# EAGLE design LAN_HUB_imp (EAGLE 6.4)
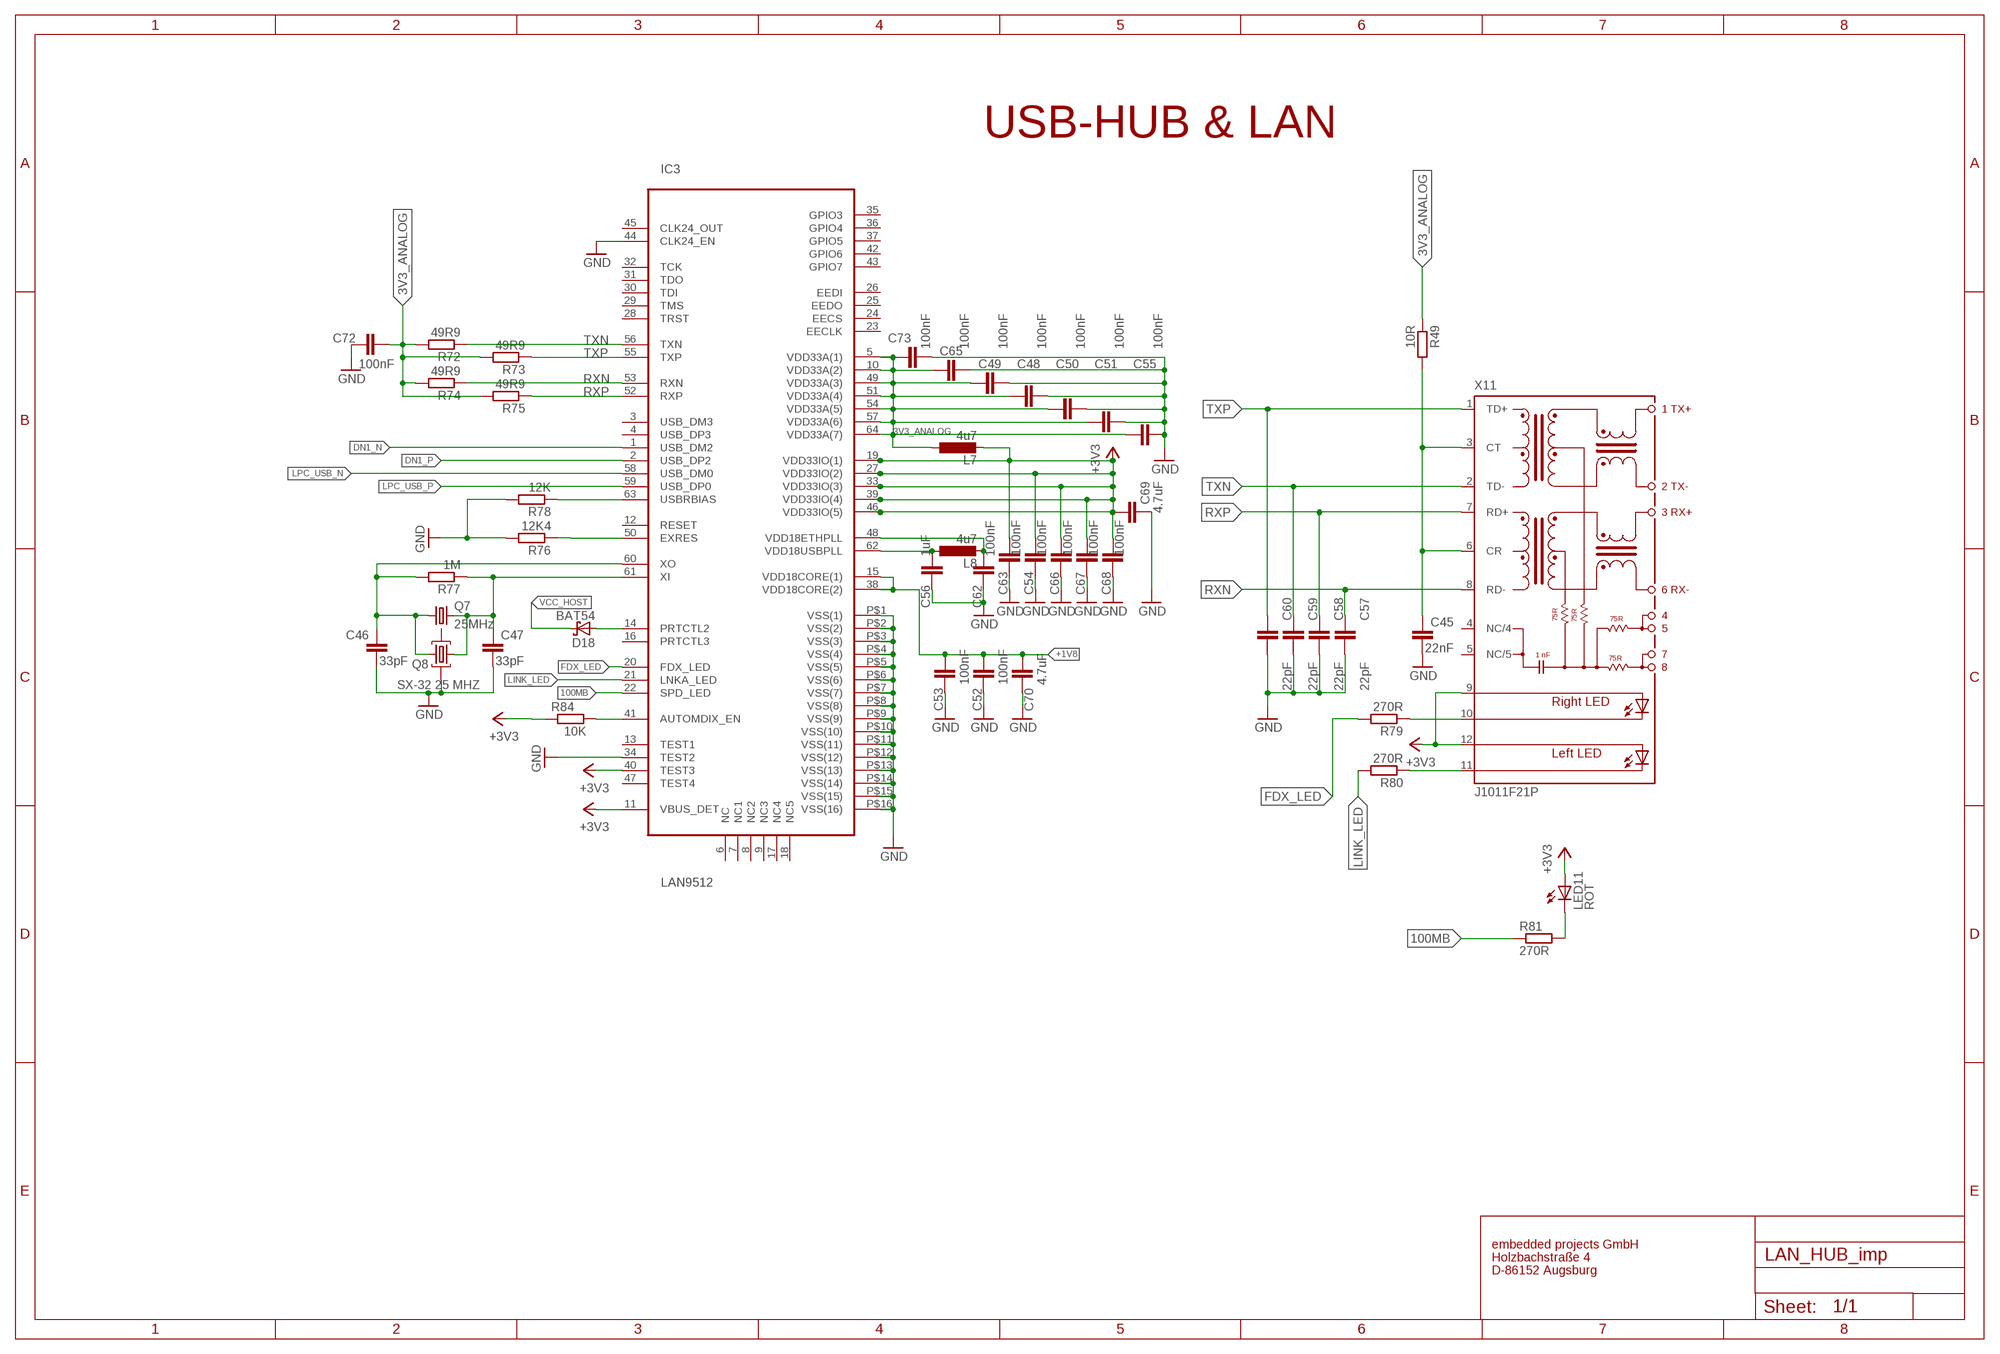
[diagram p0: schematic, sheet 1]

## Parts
C45  22nF  C-EUC0805  [C0805]
C46  33pF  C-EUC0805  [C0805]
C47  33pF  C-EUC0805  [C0805]
C48  100nF  C-EUC0805  [C0805]
C49  100nF  C-EUC0805  [C0805]
C50  100nF  C-EUC0805  [C0805]
C51  100nF  C-EUC0805  [C0805]
C52  100nF  C-EUC0805  [C0805]
C53  100nF  C-EUC0805  [C0805]
C54  100nF  C-EUC0805  [C0805]
C55  100nF  C-EUC0805  [C0805]
C56  1uF  C-EUC0805  [C0805]
C57  22pF  C-EUC0805  [C0805]
C58  22pF  C-EUC0805  [C0805]
C59  22pF  C-EUC0805  [C0805]
C60  22pF  C-EUC0805  [C0805]
C62  100nF  C-EUC0805  [C0805]
C63  100nF  C-EUC0805  [C0805]
C65  100nF  C-EUC0805  [C0805]
C66  100nF  C-EUC0805  [C0805]
C67  100nF  C-EUC0805  [C0805]
C68  100nF  C-EUC0805  [C0805]
C69  4.7uF  C-EUC0805  [C0805]
C70  4.7uF  C-EUC0805  [C0805]
C72  100nF  C-EUC0805  [C0805]
C73  100nF  C-EUC0805  [C0805]
D18  BAT54  DIODE_BAT54  [SOT-23]
IC3  LAN9512  [QFN-64]
L7  4u7  PSU3014  [PSU3014]
L8  4u7  PSU3014  [PSU3014]
LED11  ROT  LED_LEDCHIPLED_0805  [LED_CHIP-LED0805]
Q7  25MHz  CRYSTALHC49UP  [HC49UP]
Q8  SX-32 25 MHZ  SX-32  [SX-32]
R49  10R  R-EU_R0805  [R0805]
R72  49R9  R-EU_R0805  [R0805]
R73  49R9  R-EU_R0805  [R0805]
R74  49R9  R-EU_R0805  [R0805]
R75  49R9  R-EU_R0805  [R0805]
R76  12K4  R-EU_R0805  [R0805]
R77  1M  R-EU_R0805  [R0805]
R78  12K  R-EU_R0805  [R0805]
R79  270R  R-EU_R0805  [R0805]
R80  270R  R-EU_R0805  [R0805]
R81  270R  R-EU_R0805  [R0805]
R84  10K  R-EU_R0805  [R0805]
X11  J1011F21P  [J1]

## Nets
3V3_ANALOG: C48.2 C49.2 C50.2 C51.2 C55.2 C65.2 C72.1 C73.2 IC3.5(VDD33A(1)) IC3.10(VDD33A(2)) IC3.49(VDD33A(3)) IC3.51(VDD33A(4)) IC3.54(VDD33A(5)) IC3.57(VDD33A(6)) IC3.64(VDD33A(7)) L7.2 R49.1 R72.2 R73.2 R74.2 R75.2
100MB: IC3.22(SPD_LED) R81.1
+1V8: C52.2 C53.2 C70.1 IC3.15(VDD18CORE(1)) IC3.38(VDD18CORE(2))
+3V3: C54.2 C63.2 C66.2 C67.2 C68.2 C69.2 IC3.11(VBUS_DET) IC3.19(VDD33IO(1)) IC3.27(VDD33IO(2)) IC3.33(VDD33IO(3)) IC3.39(VDD33IO(4)) IC3.40(TEST3) IC3.46(VDD33IO(5)) L7.1 LED11.A R84.1 X11.9(A-R) X11.12(AL)
DN1_N: IC3.1(USB_DM2)
DN1_P: IC3.2(USB_DP2)
FDX_LED: IC3.20(FDX_LED) R79.2
GND: C45.1 C46.1 C47.1 C48.1 C49.1 C50.1 C51.1 C52.1 C53.1 C54.1 C55.1 C56.2 C57.1 C58.1 C59.1 C60.1 C62.2 C63.1 C65.1 C66.1 C67.1 C68.1 C69.1 C70.2 C72.2 C73.1 IC3.34(TEST2) IC3.44(CLK24_EN) IC3.P$1(VSS(1)) IC3.P$2(VSS(2)) IC3.P$3(VSS(3)) IC3.P$4(VSS(4)) IC3.P$5(VSS(5)) IC3.P$6(VSS(6)) IC3.P$7(VSS(7)) IC3.P$8(VSS(8)) IC3.P$9(VSS(9)) IC3.P$10(VSS(10)) IC3.P$11(VSS(11)) IC3.P$12(VSS(12)) IC3.P$13(VSS(13)) IC3.P$14(VSS(14)) IC3.P$15(VSS(15)) IC3.P$16(VSS(16)) Q8.2 R76.2 R78.2
LINK_LED: IC3.21(LNKA_LED) R80.2
LPC_USB_N: IC3.58(USB_DM0)
LPC_USB_P: IC3.59(USB_DP0)
N$10: C56.1 IC3.62(VDD18USBPLL) L8.2
N$11: LED11.C R81.2
N$21: C45.2 R49.2 X11.3(CT) X11.6(CR)
N$22: IC3.50(EXRES) R76.1
N$42: C62.1 IC3.48(VDD18ETHPLL) L8.1
N$61: C46.2 IC3.60(XO) Q7.1 Q8.3 R77.2
N$63: C47.2 IC3.61(XI) Q7.2 Q8.1 R77.1
N$65: IC3.63(USBRBIAS) R78.1
N$68: R79.1 X11.10(C-R)
N$76: R80.1 X11.11(C-L)
N$77: IC3.41(AUTOMDIX_EN) R84.2
N$78: D18.1(A) IC3.14(PRTCTL2)
RXN: C57.2 IC3.53(RXN) R74.1 X11.8(RD-)
RXP: C58.2 IC3.52(RXP) R75.1 X11.7(RD+)
TXN: C59.2 IC3.56(TXN) R72.1 X11.2(TD-)
TXP: C60.2 IC3.55(TXP) R73.1 X11.1(TD+)
VCC_HOST: D18.3(C)
Unconnected: IC3.3(USB_DM3) IC3.4(USB_DP3) IC3.6(NC) IC3.7(NC1) IC3.8(NC2) IC3.9(NC3) IC3.12(RESET) IC3.13(TEST1) IC3.16(PRTCTL3) IC3.17(NC4) IC3.18(NC5) IC3.23(EECLK) IC3.24(EECS) IC3.25(EEDO) IC3.26(EEDI) IC3.28(TRST) IC3.29(TMS) IC3.30(TDI) IC3.31(TDO) IC3.32(TCK) IC3.35(GPIO3) IC3.36(GPIO4) IC3.37(GPIO5) IC3.42(GPIO6) IC3.43(GPIO7) IC3.45(CLK24_OUT) IC3.47(TEST4) Q8.4 X11.4(NC/4) X11.5(NC/5)

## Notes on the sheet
- USB-HUB & LAN
- embedded projects GmbH
- Holzbachstraße 4
- D-86152 Augsburg

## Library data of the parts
C45-C60 C62 C63 C65-C70 C72 C73 = rcl:C-EU: CAPACITOR, European symbol
D18 = EmbeddedProjectsBauteile:DIODE_BAT54: Schottky Diodes; EP: 400113
IC3 = EmbeddedProjectsBauteile:LAN9512: USB 2.0 Hub and 10/100 Ethernet Controller; FARNELL: 2292586
L7 L8 = KUBUS3B_PARTS2:PSU3014: SMD Power Inductors Shielded
LED11 = EmbeddedProjectsBauteile:LED_LED
Q7 = crystal:CRYSTAL: CRYSTAL; OC_FARNELL: unknown; OC_NEWARK: unknown
Q8 = KUBUS3B_PARTS2:SX-32: SMD CRYSTAL; FARNELL: 1712841
R49 R72-R81 R84 = rcl:R-EU_: RESISTOR, European symbol
X11 = con-pulse:J1011F: PULSEJACK (TM) 1x1 Tab-UP RJ45 10/100 Base-TX RJ45 1x1 Tab-UP with LEDs 8-pin (J1 series) and 6-pin (JP series) integrated magnetics connector, designed to support applications, such as ADSL modems, LAN-on-Motherboard, and Hub and Switches. Source: www.pulseeng.com .. PulseJack-J402.pdf; OC_FARNELL: unknown; OC_NEWARK: unknown

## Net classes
0 default: clearance 0.15 mm
1 USB5V_EXT: width 0.15 mm, drill 0.3 mm, clearance 0.15 mm
2 5V: width 0.2 mm, clearance 0.15 mm
3 RELAY: width 1 mm, clearance 0.5 mm
5 0.15: width 0.125 mm, drill 0.3 mm, clearance 0.15 mm

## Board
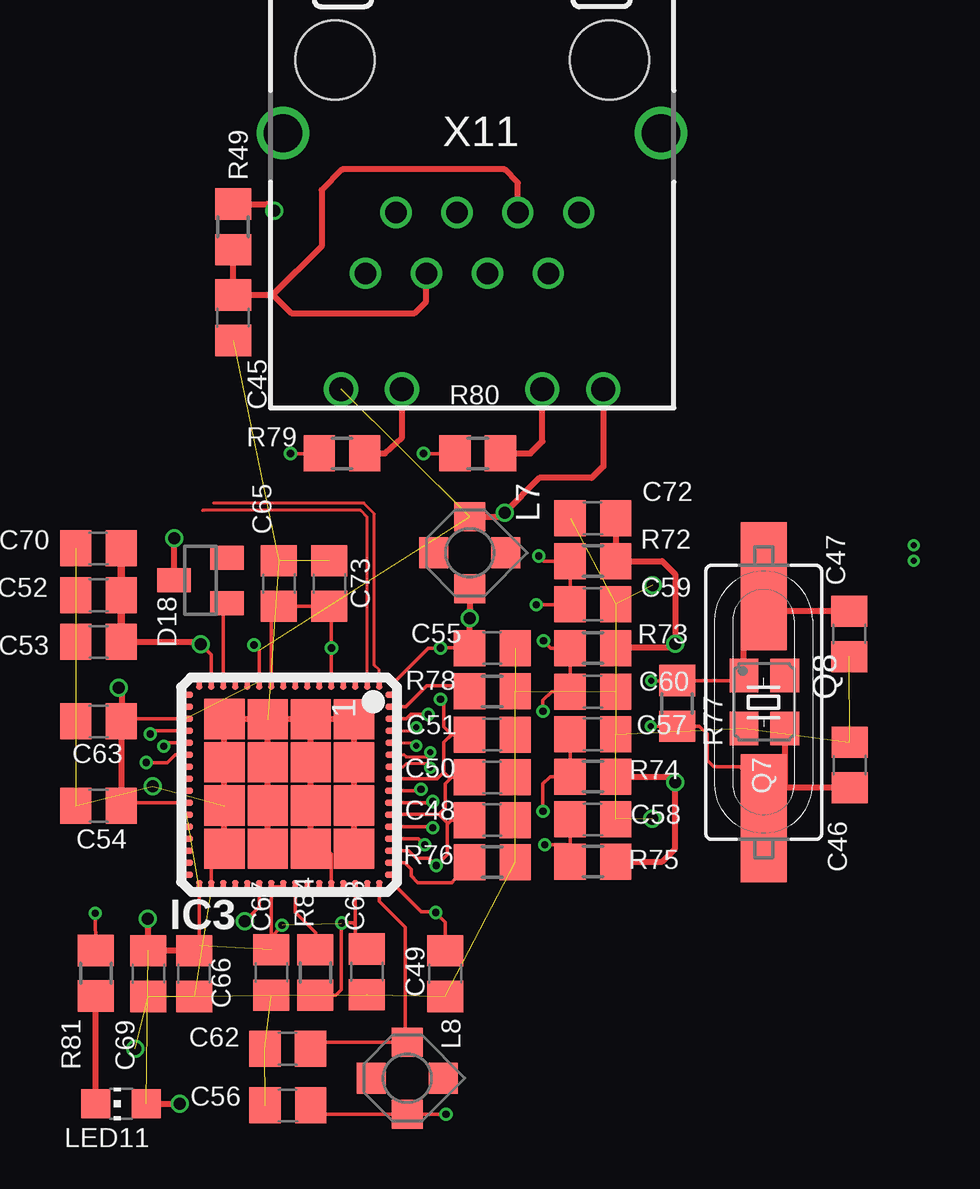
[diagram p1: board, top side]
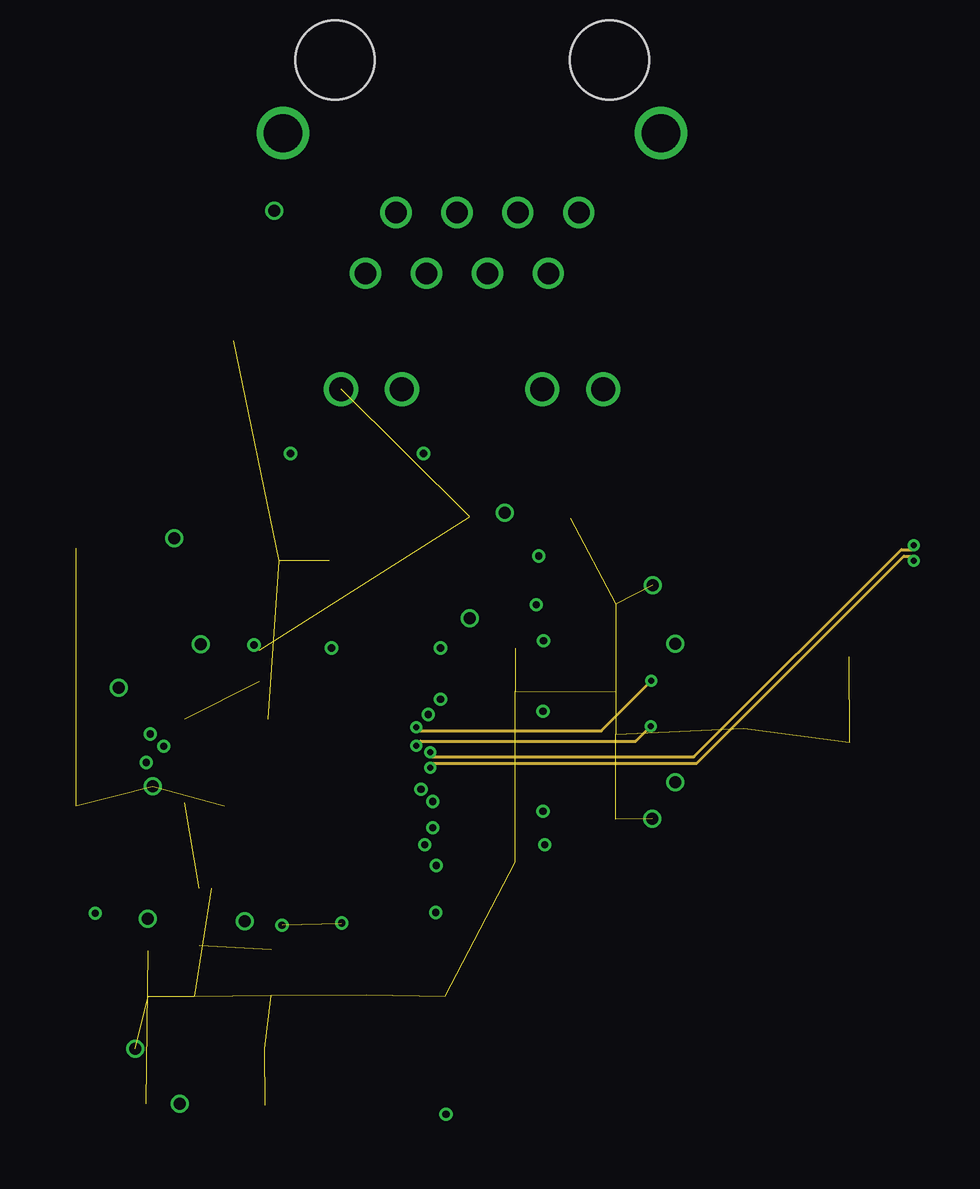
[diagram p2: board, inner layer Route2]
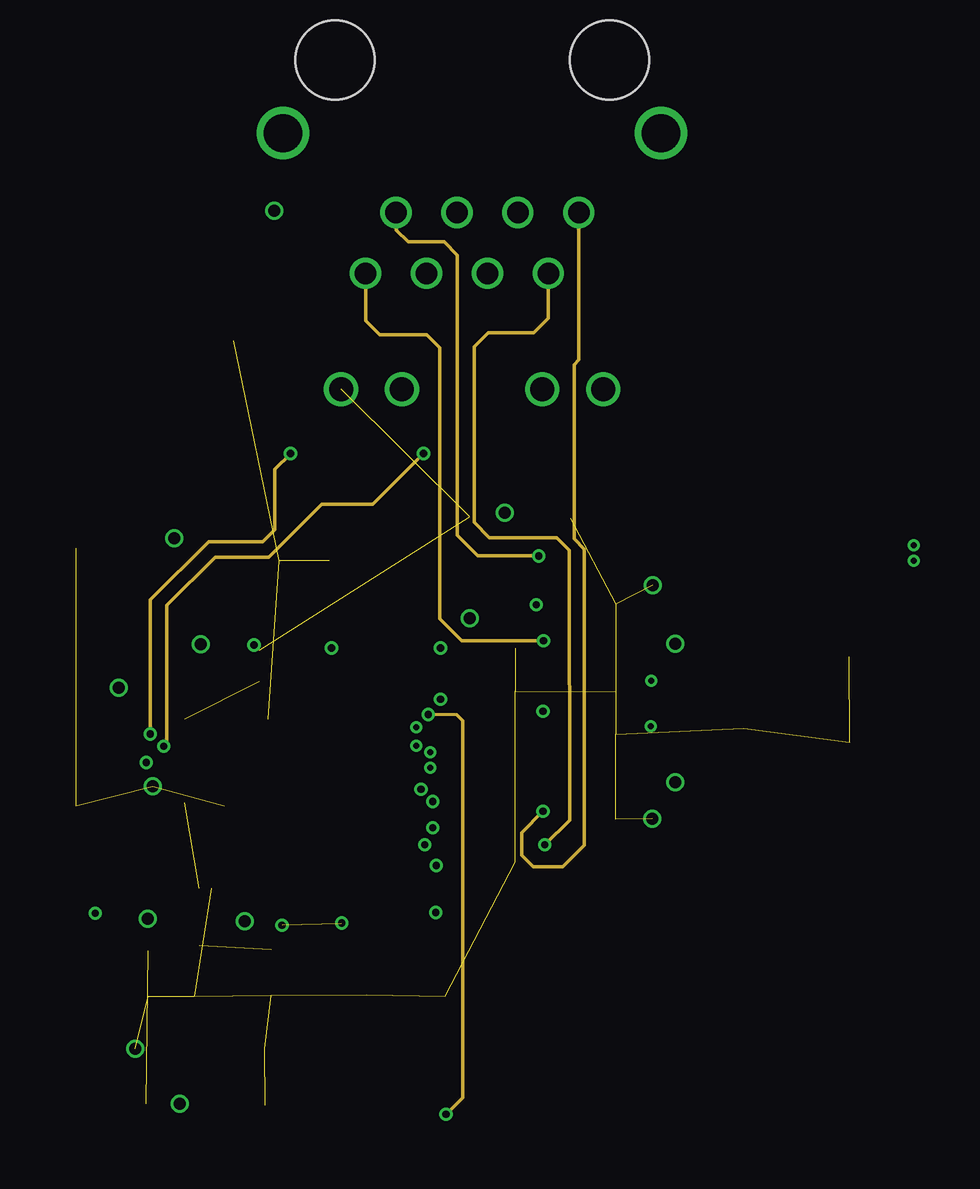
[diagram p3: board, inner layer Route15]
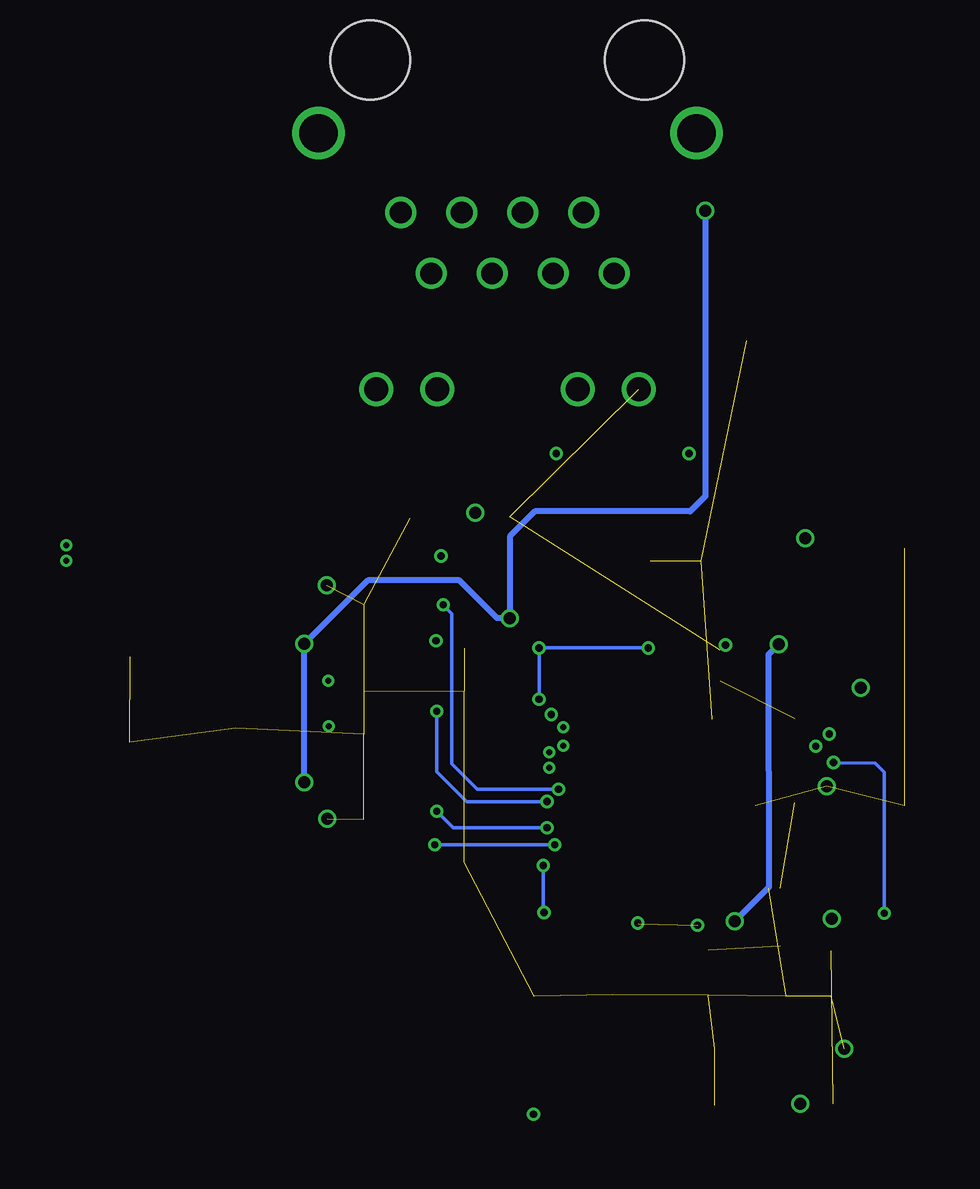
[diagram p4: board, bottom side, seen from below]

No outline drawn. Coordinates in mm, seen from the top.
Copper layers (1*2+15*16): Top 0.012mm / dielectric 0.36mm / Route2 0.018mm / dielectric 0.71mm / Route15 0.035mm / dielectric 0.2mm / Bottom 0.012mm
Design rules "125um_0.2mmborhung_4Layer *": minimum track width 0.125mm, minimum drill 0.25mm, track to track 0.125mm, track to pad 0.125mm, pad to pad 0.125mm, via to via 0.125mm, smd to smd 0mil, copper to edge 0.45mm, drill to drill 0.3mm, minimum pad ring 0.125mm, minimum via ring 0.125mm, stop-mask expansion 0.1mm, vias tented up to drill 40mil, thermal gap 0.2mm

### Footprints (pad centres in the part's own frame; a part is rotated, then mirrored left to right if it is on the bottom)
C0805 = smd 1.3 x 1.5: 1 -0.95,0; 2 0.95,0
SOT-23 = smd 1 x 1.4: 1 -0.95,-1.1; 2 0.95,-1.1; 3 0,1.1
QFN-64 = smd 0.27 x 0.7: 1 0.98,0.42; 2 1.48,0.42; 3 1.98,0.42; 4 2.48,0.42; 5 2.98,0.42; 6 3.48,0.42; 7 3.98,0.42; 8 4.48,0.42; 9 4.98,0.42; 10 5.48,0.42; 11 5.98,0.42; 12 6.48,0.42; 13 6.98,0.42; 14 7.48,0.42; 15 7.98,0.42; 16 8.48,0.42; 33 8.48,9.05; 34 7.98,9.05; 35 7.48,9.05; 36 6.98,9.05; 37 6.48,9.05; 38 5.98,9.05; 39 5.48,9.05; 40 4.98,9.05; 41 4.48,9.05; 42 3.98,9.05; 43 3.48,9.05; 44 2.98,9.05; 45 2.48,9.05; 46 1.98,9.05; 47 1.48,9.05; 48 0.98,9.05 | smd 0.7 x 0.27: 17 9.08,0.98; 18 9.08,1.48; 19 9.08,1.98; 20 9.08,2.48; 21 9.08,2.98; 22 9.08,3.48; 23 9.08,3.98; 24 9.08,4.48; 25 9.08,6.48; 26 9.08,5.98; 27 9.08,5.48; 28 9.08,4.98; 29 9.08,6.98; 30 9.08,7.48; 31 9.08,7.98; 32 9.08,8.48; 49 0.39,8.48; 50 0.39,7.98; 51 0.39,7.48; 52 0.39,6.98; 53 0.39,6.48; 54 0.39,5.98; 55 0.39,5.48; 56 0.39,4.98; 57 0.38,4.48; 58 0.38,3.98; 59 0.38,3.48; 60 0.38,2.98; 61 0.38,2.48; 62 0.38,1.98; 63 0.38,1.48; 64 0.38,0.98 | smd 1.676 x 1.676: P$1 2.03,2; P$2 3.83,2; P$3 5.63,2; P$4 7.43,1.99; P$5 7.43,3.8; P$6 5.63,3.8; P$7 3.83,3.8; P$8 2.03,3.8; P$9 2.03,5.6; P$10 3.83,5.6; P$11 5.63,5.6; P$12 7.43,5.6; P$13 7.43,7.4; P$14 5.63,7.4; P$15 3.83,7.4; P$16 2.03,7.4
PSU3014 = smd 1.2 x 1.3: 1 -1.5,0; 2 1.5,0 | smd 1.3 x 1.2: 3 0,1.5; 4 0,-1.5
LED_CHIP-LED0805 = smd 1.2 x 1.2: A 0,-1.05; C 0,1.05
HC49UP = smd 5.334 x 1.93: 1 -4.826,0; 2 4.826,0
SX-32 = smd 1.4 x 1.2: 1 -1.1,-0.85; 2 1.1,-0.85; 3 1.1,0.85; 4 -1.1,0.85
R0805 = smd 1.3 x 1.5: 1 -0.95,0; 2 0.95,0
J1 = drill 0.9 pad 1.3: 1 4.445,2.54; 2 3.175,0; 3 1.905,2.54; 4 0.635,0; 5 -0.635,2.54; 6 -1.905,0; 7 -3.175,2.54; 8 -4.445,0 | drill 1 pad 1.422: 9 5.465,7.37; 10 2.925,7.37; 11 -2.925,7.37; 12 -5.465,7.37 | drill 1.6 pad 2.184: M1 -7.875,-3.3; M2 7.875,-3.3 | hole 3.3: 5.715,-6.35; -5.715,-6.35

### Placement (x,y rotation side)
C45  8.35,50.03 90 top
C46  34.04,31.39 270 top
C47  34.02,36.85 90 top
C48  19.15,29.1 180 top
C49  17.19,22.7 90 top
C50  19.15,30.88 180 top
C51  19.15,32.66 180 top
C52  2.74,38.47 0 top
C53  2.74,36.52 0 top
C54  2.74,29.7 0 top
C55  19.15,36.27 180 top
C56  10.63,17.21 180 top
C57  23.34,32.68 180 top
C58  23.34,29.13 180 top
C59  23.34,38.09 180 top
C60  23.34,34.45 180 top
C62  10.62,19.57 180 top
C63  2.74,33.21 0 top
C65  10.26,38.96 270 top
C66  6.72,22.7 90 top
C67  9.94,22.75 90 top
C68  13.92,22.78 90 top
C69  4.82,22.7 90 top
C70  2.74,40.42 180 top
C72  23.34,41.68 180 top
C73  12.36,38.96 270 top
D18  6.99,39.09 90 top
IC3  15.42,35.31 180 top
L7  18.21,40.23 270 top
L8  15.61,18.35 270 top
LED11  3.68,17.28 90 top
Q7  30.46,34.01 90 top
Q8  30.48,34.02 270 top
R49  8.35,53.82 270 top
R72  23.34,39.89 0 top
R73  23.34,36.27 0 top
R74  23.34,30.91 0 top
R75  23.34,27.37 0 top
R76  19.15,27.35 0 top
R77  26.85,33.96 270 top
R78  19.15,34.46 0 top
R79  12.89,44.38 180 top
R80  18.54,44.38 180 top
R81  2.63,22.72 270 top
R84  11.77,22.75 90 top
X11  18.31,54.42 180 top

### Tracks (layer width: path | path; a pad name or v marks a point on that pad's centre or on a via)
3V3_ANALOG  (via drill 0.3, 0.5)
  Top 0.15: C48.2 17.44,29.1 17.27,28.93 | 17.27,28.93 17.27,27.66 16.89,27.28 v16.82,27.2 16.51,27.51 15.98,27.51 15.67,27.81 15.04,27.81 IC3.51 | C50.2 17.47,30.88 | 17.47,30.88 17.2,30.61 17.2,29.62 16.92,29.34 | 16.92,29.34 IC3.54 | C51.2 17.45,32.66 17.12,32.33 | 17.12,32.33 17.12,31.09 | 17.12,31.09 16.86,30.83 IC3.57 | IC3.49 15.03,26.45 16.18,25.27 16.76,25.27 v16.79,25.25 17.2,24.84 C49.2 | 17.27,28.93 17.27,28.98 16.92,29.34 | 17.47,30.88 17.33,30.88 17.12,31.09 | IC3.64 15.06,34.35 15.06,34.85 16.48,36.27 v16.99,36.27 C55.2 | 17.12,32.33 17.45,32.66 17.12,32.99 17.12,34.01 v16.99,34.14 | IC3.5 12.44,36.26 v12.45,36.27 12.44,36.3 12.44,37.93 C73.2 12.34,38.01 C65.2 9.94,37.74 IC3.10
  Top 0.254: R75.2 26.23,27.37 26.77,27.91 26.77,30.63 v26.77,30.68 26.55,30.91 R74.2 | R73.2 26.59,36.27 v26.77,36.45 26.77,39.34 26.23,39.89 R72.2 C72.1 | C55.2 18.2,37.5 v18.21,37.52 18.21,37.54 L7.2 | R49.1 9.77,54.77 v10.06,54.48
  Bottom 0.15: v16.99,34.14 v16.99,36.27 16.23,36.27 v12.45,36.27 | v16.82,27.2 16.82,25.27 v16.79,25.25
  Bottom 0.254: v26.77,30.68 v26.77,36.45 24.13,39.09 20.32,39.09 18.74,37.52 v18.21,37.52 18.21,40.92 17.17,41.96 10.69,41.96 10.06,42.6 v10.06,54.48
100MB  (via drill 0.3)
  Top 0.15: IC3.22 5.94,31.83 5.61,31.5 v4.72,31.5 | v2.61,25.22 2.63,23.72 R81.1
  Bottom 0.15: v4.72,31.5 2.99,31.48 2.61,31.09 v2.61,25.22
+1V8  (via drill 0.5)
  Top 0.15: IC3.38 9.44,25.49 v8.84,24.89 | IC3.15 7.44,36 v7.01,36.42
  Top 0.254: C53.2 6.91,36.52 v7.01,36.42
  Top 0.305: C70.1 C52.2 C53.2
  Bottom 0.254: v7.01,36.42 7.44,35.99 7.42,26.31 v8.84,24.89
+3V3  (via drill 0.3, 0.5)  (7 unrouted)
  Top 0.15: IC3.19 3.73,33.33 C63.2 | IC3.27 3.74,29.83 C54.2 | IC3.33 6.94,23.87 C66.2 | IC3.39 9.94,24.21 | 9.94,24.21 9.94,23.68 C67.2 | IC3.46 13.44,24.71 | 13.44,24.71 13.44,24.21 C68.2 | IC3.11 9.44,36.18 v9.22,36.4 | v10.39,24.71 10.34,24.66 9.94,24.21 | 13.44,24.71 13.34,24.82 v12.88,24.82 12.85,24.79 12.85,22.02 12.63,21.8 R84.1
  Top 0.254: LED11.A 6,17.28 v6.12,17.28 | L7.1 19.48,41.73 v19.66,41.91 21.11,43.36 23.29,43.36 23.77,43.84 X11.12 | 3.73,33.33 3.73,34.48 v3.58,34.62 | C63.2 C54.2 | v4.8,24.99 4.82,24.97 C69.2 C66.2 | IC3.40 IC3.39
DN1_N
  Top 0.125: IC3.1 14.44,35.37 14.24,35.56 14.24,41.86 13.8,42.3 7.57,42.3 7.53,42.3
DN1_P
  Top 0.125: IC3.2 13.94,41.72 13.66,42 7.14,42 7.07,42
FDX_LED  (via drill 0.3)
  Top 0.15: IC3.20 5.04,32.83 v4.9,32.69 | R79.2 | v10.74,44.37 R79.2
  Route15 0.15: v4.9,32.69 4.9,38.28 7.34,40.69 9.58,40.69 10.08,41.2 10.08,43.71 v10.74,44.37
GND  (via drill 0.5)  (33 unrouted)
  Top 0.15: IC3.44 12.44,27.69 IC3.P$15 | IC3.34 7.44,27.36 IC3.P$13
  Top 0.254: IC3.P$16 IC3.P$9 IC3.P$8 IC3.P$1 IC3.P$2 | IC3.P$15 IC3.P$10 IC3.P$7 IC3.P$2 | IC3.P$14 IC3.P$11 IC3.P$6 IC3.P$3 | IC3.P$13 IC3.P$12 IC3.P$5 IC3.P$4 8,33.31 IC3.P$3 | IC3.P$2 IC3.P$3
  other vias: 25.84,38.89 25.81,29.16 4.27,19.58 5,30.5
LINK_LED  (via drill 0.3)
  Top 0.15: IC3.21 5.61,32.33 v5.46,32.18 | v16.28,44.37 17.97,44.37 R80.2
  Route15 0.15: v5.46,32.18 5.59,32.33 5.59,38.05 7.59,40.06 9.83,40.06 12.04,42.27 14.17,42.27 v16.28,44.37
LPC_USB_N  (via drill 0.25)
  Top 0.125: IC3.58 15.45,31.33 15.58,31.46 16.56,31.46 v16.56,31.27 | 36.7,40.1 v36.7,39.91
  Route2 0.125: v16.56,31.27 16.56,31.46 27.67,31.46 36.3,40.1 36.7,40.1 v36.7,39.91
LPC_USB_P  (via drill 0.25)
  Top 0.125: IC3.59 15.47,31.83 15.56,31.73 16.56,31.73 v16.56,31.92 | 36.7,40.37 v36.7,40.56
  Route2 0.125: v16.56,31.92 16.56,31.73 27.55,31.73 36.19,40.37 36.7,40.37 v36.7,40.56
N$10  (via drill 0.3)
  Top 0.15: IC3.62 15.57,33.33 15.75,33.5 v16.48,33.5 | v17.22,16.84 15.51,16.84 | 15.51,16.84 L8.2 | 15.51,16.84 11.95,16.84 C56.1
  Route15 0.15: v16.48,33.5 17.66,33.48 17.92,33.23 17.92,17.54 v17.22,16.84
N$11
  Top 0.254: LED11.C R81.2
N$21
  Top 0.254: R49.2 C45.2 10.01,50.98 | 10.01,50.98 10.78,50.22 15.91,50.22 16.39,50.7 16.4,51.74 X11.3 | X11.6 20.21,55.66 19.66,56.21 12.9,56.21 12.04,55.35 12.04,53 10.01,50.98
N$22
  Top 0.15: 17.93,27.33 R76.1 18.19,27.34 17.7,26.77 17.45,26.49 16.05,26.49 15.77,26.77 15.77,27.05 15.5,27.33 IC3.50
N$42
  Top 0.15: IC3.48 14.44,25.72 15.52,24.64 15.52,19.86 L8.1 11.7,19.84 C62.1
N$61  (via drill 0.25)
  Top 0.125: IC3.60 15.91,32.33 v15.98,32.21 | v25.76,33.02 26.67,33.02 R77.2
  Top 0.15: R77.2 27.77,33.01 28.1,32.69 28.1,31.6 28.38,31.32 29.46,31.32 30.45,30.33 Q7.1
  Top 0.254: C46.2 31.34,30.44 | 31.34,30.44 30.57,30.44 30.45,30.33 | Q8.3 31.33,30.45 31.34,30.44
  Route2 0.125: v15.98,32.21 16.15,32.38 25.12,32.38 v25.76,33.02
N$63  (via drill 0.25)
  Top 0.125: IC3.61 15.83,32.83 v15.98,32.97 | v25.78,34.9 26.66,34.9 R77.1
  Top 0.15: R77.1 29.43,34.91 Q8.1
  Top 0.254: Q8.1 29.63,37.8 | 29.63,37.8 29.63,38.01 Q7.2 | C47.2 29.64,37.8 29.63,37.8
  Route2 0.125: v15.98,32.97 16.1,32.82 23.7,32.82 v25.78,34.9
N$65
  Top 0.15: IC3.63 15.54,33.83 16.41,34.7 18.01,34.7 R78.1
N$68
  Top 0.254: R79.1 14.69,44.38 15.39,45.03 15.39,47.04 X11.10
N$76
  Top 0.254: R80.1 20.73,44.38 21.23,44.88 X11.11
N$77
  Top 0.15: IC3.41 10.94,25.26 11.79,24.41 11.79,23.66 R84.2
N$78
  Top 0.15: IC3.14 7.94,37.97 D18.1
RXN  (via drill 0.3)
  Top 0.15: IC3.53 16.61,28.83 v16.66,28.78 | v21.26,29.46 21.26,30.61 21.57,30.91 R74.1 C57.2
  Route15 0.15: X11.8 22.75,48.28 22.55,48.08 22.55,40.82 22.98,40.39 22.98,28.06 22.09,27.15 20.85,27.15 20.37,27.64 20.37,28.57 v21.26,29.46
  Bottom 0.15: v16.66,28.78 20.57,28.78 v21.26,29.46
RXP  (via drill 0.3)
  Top 0.15: IC3.52 16.07,28.33 v16.33,28.07 | v21.34,28.07 22.38,28.07 22.39,28.03 | 22.39,28.03 R75.1 | C58.2 22.39,28.49 22.39,28.03
  Route15 0.15: X11.7 21.48,50.01 20.88,49.4 18.97,49.4 18.39,48.82 18.39,41.5 19.02,40.87 21.83,40.87 22.36,40.34 22.37,29.1 v21.34,28.07
  Bottom 0.15: v16.33,28.07 v21.34,28.07
TXN  (via drill 0.3)
  Top 0.15: IC3.56 16.13,30.33 v16.18,30.38 | v20.98,38.08 22.38,38.08 C59.2 R72.1 21.3,39.89 v21.08,40.11
  Route15 0.15: v21.08,40.11 18.54,40.11 17.68,40.97 17.68,52.63 17.14,53.19 15.65,53.19 15.14,53.67 X11.2
  Bottom 0.15: v16.18,30.38 19.56,30.38 20.62,31.45 20.62,37.69 v20.98,38.08
TXP  (via drill 0.3)
  Top 0.15: IC3.55 16.62,29.83 v16.66,29.87 | v21.26,33.63 21.26,34.09 21.61,34.44 C60.2 R73.1 21.59,36.27 v21.29,36.58
  Route15 0.15: v21.29,36.58 17.88,36.58 16.97,37.49 16.97,48.78 16.96,48.78 16.41,49.33 14.45,49.33 13.87,49.91 X11.1
  Bottom 0.15: v16.66,29.87 20.02,29.87 21.26,31.11 v21.26,33.63
VCC_HOST  (via drill 0.5)
  Top 0.254: D18.3 5.89,40.83 v5.89,40.84

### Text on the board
tStop: 7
